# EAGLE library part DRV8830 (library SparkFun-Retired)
DRV8830 I2C DC Motor Driver TSSOP-10 with exposed power pad 1A current limit, 2.75V to 6.8V
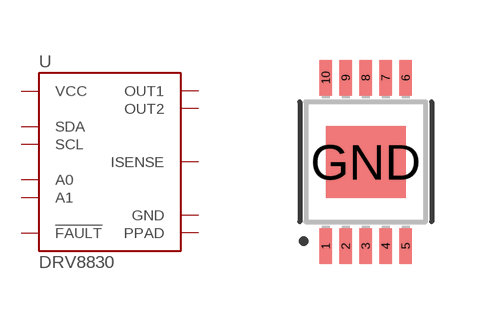
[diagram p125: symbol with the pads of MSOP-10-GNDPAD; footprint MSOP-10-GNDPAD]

Designator prefix U

## DRV8830 (PROD_ID: IC-11646)  [MSOP-10-GNDPAD]
1  OUT2  pwr
2  ISENSE
3  OUT1  pwr
4  VCC  pwr
5  GND  pwr
6  !FAULT  out
7  A0  in
8  A1  in
9  SDA
10  SCL  in
GND  PPAD  pwr

## Footprint MSOP-10-GNDPAD (pad centres in mm)
10-lead MSOP w/ center GND pad
smd 0.305 x 0.889: 1 -1,-2.11; 2 -0.5,-2.11; 3 0,-2.11; 4 0.5,-2.11; 5 1,-2.11; 6 1,2.11; 7 0.5,2.11; 8 0,2.11; 9 -0.5,2.11; 10 -1,2.11
smd 2 x 1.8: GND 0,0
